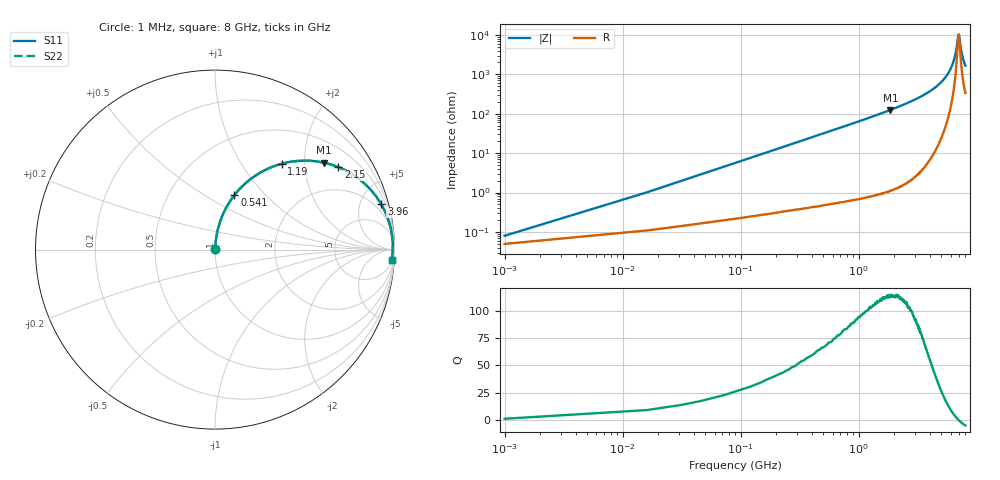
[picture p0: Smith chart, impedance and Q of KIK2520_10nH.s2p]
!version-2
!date-01.2022
!Series
# MHz S RI R 50
!Freq ReS11 ImS11 ReS21 ImS21 ReS12 ImS12 ReS22 ImS22
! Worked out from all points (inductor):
!   535 points, 1 MHz to 8 GHz, reference 50 ohm
!   read as one part in series: L = 10 nH near 31 MHz
!   highest Q = 113 at 1.85 GHz (marker M1), where L = 10.7 nH
!   self-resonance near 7.02 GHz
!   S11 on the Smith chart (normalised r, x): 1 MHz: 1.00, +0.00; 541 MHz: 1.01, +0.68; 1.19 GHz: 1.02, +1.53; 2.15 GHz: 1.03, +2.97; 3.96 GHz: 1.13, +7.30; 8 GHz: 8, -32
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1  0.000496 0.000628  0.9995 -0.000628  0.9995 -0.000628  0.000496 0.000628
46  0.00246 0.0288  0.9975 -0.0288  0.9975 -0.0288  0.00246 0.0288
76  0.00427 0.0475  0.9957 -0.0475  0.9957 -0.0475  0.00427 0.0475
121  0.00816 0.0752  0.9918 -0.0752  0.9918 -0.0752  0.00816 0.0752
196  0.0179 0.1207  0.9821 -0.1207  0.9821 -0.1207  0.0179 0.1207
286  0.0347 0.1731  0.9653 -0.1731  0.9653 -0.1731  0.0347 0.1731
541  0.1082 0.3035  0.8918 -0.3035  0.8918 -0.3035  0.1082 0.3035
826  0.2196 0.4082  0.7804 -0.4082  0.7804 -0.4082  0.2196 0.4082
1190  0.3717 0.4783  0.6283 -0.4783  0.6283 -0.4783  0.3717 0.4783
1340  0.432 0.4906  0.568 -0.4906  0.568 -0.4906  0.432 0.4906
1850  0.6074 0.4839  0.3926 -0.4839  0.3926 -0.4839  0.6074 0.4839
2150  0.6872 0.4592  0.3128 -0.4592  0.3128 -0.4592  0.6872 0.4592
2670  0.7916 0.4013  0.2084 -0.4013  0.2084 -0.4013  0.7916 0.4013
3960  0.9264 0.2524  0.0736 -0.2524  0.0736 -0.2524  0.9264 0.2524
4010  0.9291 0.2476  0.0709 -0.2476  0.0709 -0.2476  0.9291 0.2476
5340  0.9784 0.122  0.0216 -0.122  0.0216 -0.122  0.9784 0.122
6170  0.9888 0.0579  0.0112 -0.0579  0.0112 -0.0579  0.9888 0.0579
6680  0.9906 0.0225  0.00939 -0.0225  0.00939 -0.0225  0.9906 0.0225
6930  0.9905 0.00578  0.00948 -0.00578  0.00948 -0.00578  0.9905 0.00578
7040  0.9903 -0.000895  0.00969 0.000895  0.00969 0.000895  0.9903 -0.000895
7470  0.9885 -0.0275  0.0115 0.0275  0.0115 0.0275  0.9885 -0.0275
8000  0.9845 -0.0575  0.0155 0.0575  0.0155 0.0575  0.9845 -0.0575
